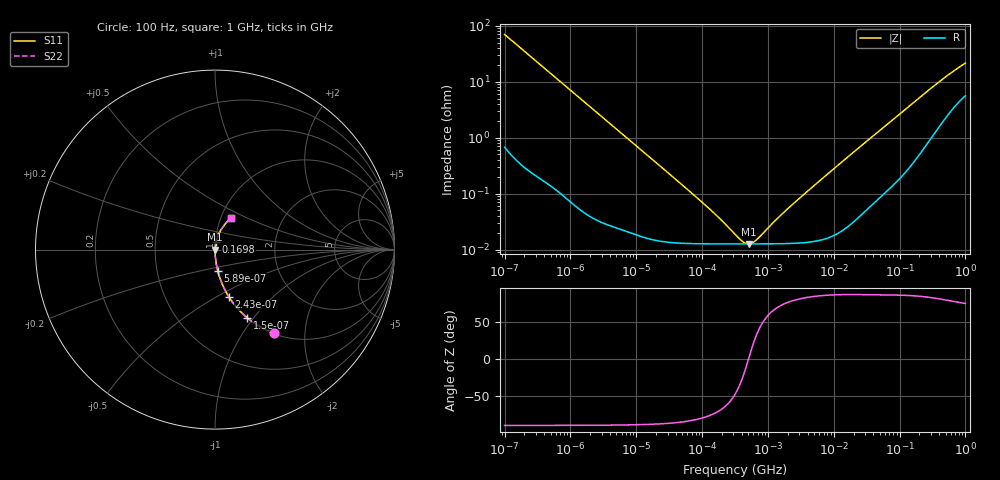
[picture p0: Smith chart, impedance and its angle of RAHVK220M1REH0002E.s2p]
! RAHVK220M1REH0002E  S-PARAMETER MODEL  (AEC-Q200 qualified)
! Model Generated by ELNA Corporation (http://www.ty-top.com)
! Version 1.0
! ELNA Control No. 201214
! Copyright (c) 2020 ELNA CO.,LTD. All Rights Reserved.
! Products Name : CONDUCTIVE POLYMER HYBRID ALUMINUM ELECTROLYTIC CAPACITORS
! Characteristics :
!  Capacitance  :  22uF  ,  Rated voltage  :  80V
!  Operating Temp. Range  :  -55 to +125 degC  ,  Endurance  :  4000hr at 125 degC
!  Dimension D  :  8mm  ,  Dimension L  :  10mm
! Frequency Range : 100Hz - 1GHz
! External Node Assignments :
!  1  o---| |---o  2
# MHz S RI R 50
!Freq[MHz].  S11 Real  S11 Imag  S21 Real  S21 Imag  S12 Real  S12 Imag  S22 Real  S22 Imag
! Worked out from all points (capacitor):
!   401 points, 100 Hz to 1 GHz, reference 50 ohm
!   read as one part in series: C = 22.8 uF near 108 Hz
!   lowest |Z| = 12.6 mohm at 512.9 kHz (marker M1)
!   series resonance near 507.5 kHz, so ESL is about 4.3 nH
!   S11 on the Smith chart (normalised r, x): 100 Hz: 1.01, -1.39; 150 Hz: 1.01, -0.93; 243 Hz: 1.00, -0.58; 589 Hz: 1.00, -0.24; 169.8 MHz: 1.01, +0.09; 1 GHz: 1.11, +0.41
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0.0001  0.3287 -0.4649  0.6713 0.4649  0.6713 0.4649  0.3287 -0.4649
0.00015  0.1806 -0.3805  0.8194 0.3805  0.8194 0.3805  0.1806 -0.3805
0.000243  0.0784 -0.2646  0.9216 0.2646  0.9216 0.2646  0.0784 -0.2646
0.000378  0.0347 -0.1784  0.9653 0.1784  0.9653 0.1784  0.0347 -0.1784
0.000589  0.0151 -0.1172  0.9849 0.1172  0.9849 0.1172  0.0151 -0.1172
0.001488  0.00273 -0.0473  0.9973 0.0473  0.9973 0.0473  0.00273 -0.0473
0.004241  0.000538 -0.0167  0.9995 0.0167  0.9995 0.0167  0.000538 -0.0167
0.022131  0.000152 -0.00323  0.9998 0.00323  0.9998 0.00323  0.000152 -0.00323
0.12517  0.000127 -0.000538  0.9999 0.000538  0.9999 0.000538  0.000127 -0.000538
0.203002  0.000126 -0.000296  0.9999 0.000296  0.9999 0.000296  0.000126 -0.000296
0.316228  0.000126 -0.000139  0.9999 0.000139  0.9999 0.000139  0.000126 -0.000139
0.419276  0.000126 -5.42e-05  0.9999 5.42e-05  0.9999 5.42e-05  0.000126 -5.42e-05
0.512861  0.000126 3.01e-06  0.9999 -3.01e-06  0.9999 -3.01e-06  0.000126 3.01e-06
0.578762  0.000126 3.73e-05  0.9999 -3.73e-05  0.9999 -3.73e-05  0.000126 3.73e-05
0.679986  0.000126 8.39e-05  0.9999 -8.39e-05  0.9999 -8.39e-05  0.000126 8.39e-05
1.650061  0.000127 0.000416  0.9999 -0.000416  0.9999 -0.000416  0.000127 0.000416
4.704354  0.000139 0.00129  0.9999 -0.00129  0.9999 -0.00129  0.000139 0.00129
69.9842  0.00155 0.0184  0.9984 -0.0184  0.9984 -0.0184  0.00155 0.0184
169.8244  0.00572 0.0434  0.9943 -0.0434  0.9943 -0.0434  0.00572 0.0434
484.1724  0.0334 0.1102  0.9666 -0.1102  0.9666 -0.1102  0.0334 0.1102
754.2234  0.0631 0.1508  0.9369 -0.1508  0.9369 -0.1508  0.0631 0.1508
1000  0.0881 0.1787  0.9119 -0.1787  0.9119 -0.1787  0.0881 0.1787
